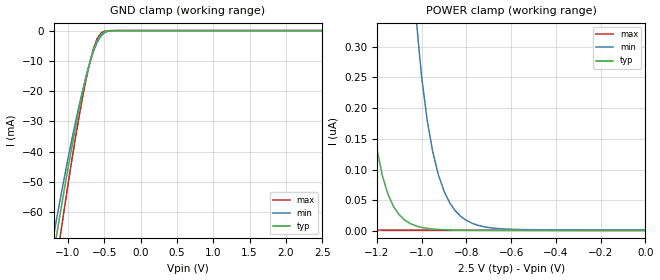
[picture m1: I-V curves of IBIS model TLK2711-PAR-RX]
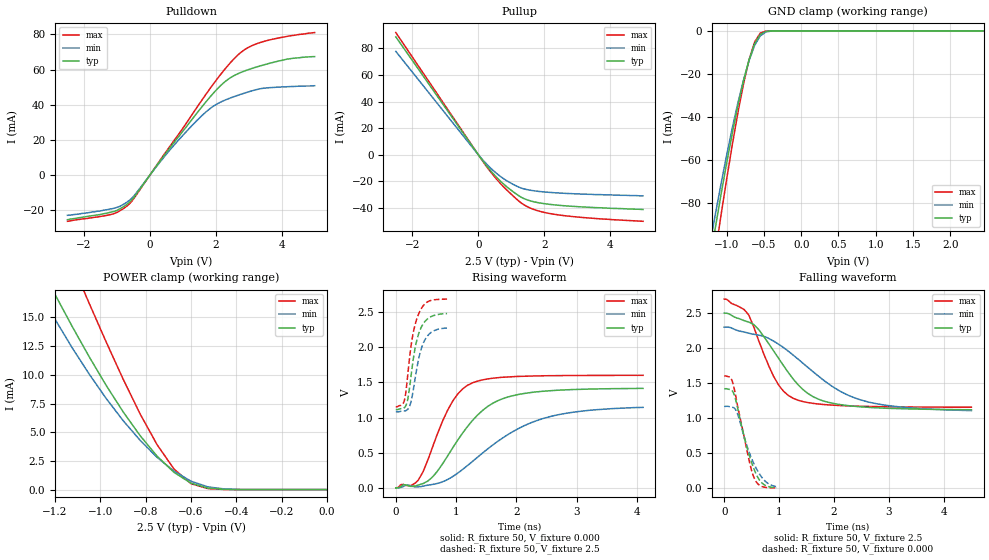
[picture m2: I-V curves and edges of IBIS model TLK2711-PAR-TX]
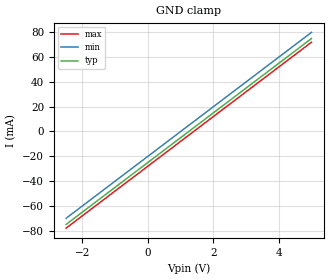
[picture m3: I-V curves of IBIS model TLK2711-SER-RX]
[IBIS ver]   3.2
[File name]   tlk2711.ibs
[File Rev]   0
[Date]   05/17/2001
[Source]   TI
[Notes]   This model is for the TLK2711/TLK2711A SerDes device
[Copyright]   Copyright 2001 Mentor Graphics, Inc.
| (C) COPYRIGHT 1993-2001
| MENTOR GRAPHICS CORPORATION
| ICX STANDARD LIBRARY, ICX PROJECT MODELING,
| ICX CUSTOM MODELING, ICX VENDOR MODEL
| ALL RIGHTS RESERVED.
| THE FOLLOWING ARE TRADEMARKS OR SERVICE MARKS OF
| MENTOR GRAPHICS CORPORATION:ICX (R), ICX STANDARD
| LIBRARY(R), ICX PROJECT MODELING(R), ICX CUSTOM
| MODELING(R), qualityIBIS(TM), MODELVIEWER(TM),  AND MODELEDITOR(TM).
| ALL COPIES OF SOFTWARE, INCLUDING BUT NOT LIMITED TO
| ANY MODIFICATIONS, ENHANCEMENTS OR DERIVATIVE
| WORKS, MUST CONTAIN ALL MENTOR GRAPHICS
| CORPORATION'S NOTICES AND LEGENDS, INCLUDING
| THOSE EMBEDDED IN SOFTWARE AND THOSE AFFIXED
| TO SOFTWARE MEDIUM AND CONTAINER, AS RECEIVED
| FROM MENTOR GRAPHICS CORPORATION
| ALL OTHER BRANDS AND PRODUCT NAMES ARE
| TRADEMARKS OF THEIR RESPECTIVE OWNERS.
| LICENSED SOFTWARE IS THE LICENSE TO USE THE
| ICX STANDARD LIBRARY ICX PROJECT MODELING
| ICX CUSTOM MODELING ICX VENDOR MODEL
|   Component TLK2711
[Component]   TLK2711
[Manufacturer]  TI
[Package]
| variable   typ   min   max
R_pkg   0.0m   0.0m   0.0m
L_pkg   0.0nH   0.0nH   0.0nH
C_pkg   0.0pF   0.0pF   0.0pf
[Pin]   signal_name   model_name   R_pin   L_pin   C_pin
1   VDD   POWER
2   TXD3   TLK2711-PAR-RX
3   TXD4   TLK2711-PAR-RX
4   TXD5   TLK2711-PAR-RX
5   GND   GND
6   TXD6   TLK2711-PAR-RX
7   TXD7   TLK2711-PAR-RX
8   GTX_CLK   TLK2711-PAR-RX
9   VDD   POWER
10   TXD8   TLK2711-PAR-RX
11   TXD9   TLK2711-PAR-RX
12   TXD10   TLK2711-PAR-RX
13   GND   GND
14   TXD11   TLK2711-PAR-RX
15   TXD12   TLK2711-PAR-RX
16   TXD13   TLK2711-PAR-RX
17   TXD14   TLK2711-PAR-RX
18   GND   GND
19   TXD15   TLK2711-PAR-RX
20   TKMSB   TLK2711-PAR-RX
21   LOOPEN   TLK2711-PAR-RX
22   TKLSB   TLK2711-PAR-RX
23   VDD   POWER
24   ENABLE   TLK2711-PAR-RX
25   LCKREFN   TLK2711-PAR-RX
26   PRBSEN   TLK2711-PAR-RX
27   TESTEN   TLK2711-PAR-RX
28   GND   GND
29   RKLSB   TLK2711-PAR-TX
30   RKMSB   TLK2711-PAR-TX
31   RXD15   TLK2711-PAR-TX
32   RXD14   TLK2711-PAR-TX
33   GND   GND
34   RXD13   TLK2711-PAR-TX
35   RXD12   TLK2711-PAR-TX
36   RXD11   TLK2711-PAR-TX
37   RXD10   TLK2711-PAR-TX
38   VDD   POWER
39   RXD9   TLK2711-PAR-TX
40   RXD8   TLK2711-PAR-TX
41   RX_CLK   TLK2711-PAR-TX
42   RXD7   TLK2711-PAR-TX
43   GND   GND
44   RXD6   TLK2711-PAR-TX
45   RXD5   TLK2711-PAR-TX
46   RXD4   TLK2711-PAR-TX
47   RXD3   TLK2711-PAR-TX
48   VDD   POWER
49   RXD2   TLK2711-PAR-TX
50   RXD1   TLK2711-PAR-TX
51   RXD0   TLK2711-PAR-TX
52   GNDA   GND
53   DINRXN   TLK2711-SER-RX
54   DINRXP   TLK2711-SER-RX
55   VDDA   POWER
56   PRE   TLK2711-PAR-RX
57   VDDA   POWER
58   GNDA   GND
59   DOUTTXN   TLK2711-SER-TX
60   DOUTTXP   TLK2711-SER-TX
61   GNDA   GND
62   TXD0   TLK2711-PAR-RX
63   TXD1   TLK2711-PAR-RX
64   TXD2   TLK2711-PAR-RX
[Diff Pin]   inv_pin   vdiff   tdelay_typ tdelay_min tdelay_max
  54   53   200mV   NA   NA   NA
  60   59   1200mV   NA   NA   NA
[Model selector]   TLK2711-SER-TX
TLK2711-SER-TX_05  TLK2711-SER-TX_05
TLK2711-SER-TX_20  TLK2711-SER-TX_20
| Models and submodels in the file (5): TLK2711-PAR-RX (Input), TLK2711-PAR-TX (3-state), TLK2711-SER-RX (Input), TLK2711-SER-TX_05 (3-state), TLK2711-SER-TX_20 (3-state)
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|   Model TLK2711-PAR-RX
[Model]   TLK2711-PAR-RX
Model_type   Input
Polarity   Non-Inverting
Vinl = 0.8
Vinh = 1.7
| C_comp is estimated by modeling group by simulation
C_comp   3.7441pF   3.6871pF   4.0174pF
[Temperature Range]   27   85   -40
[Voltage Range]   2.5V   2.3V   2.7V
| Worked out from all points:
|   GND clamp passes 1 mA (typ) near -0.53 V on its own axis
[GND_clamp]
| voltage   I(typ)   I(min)   I(max)
-2.5V     -288.4mA   -250.7mA   -333.7mA
-1.2V     -74mA      -67.93mA   -83.57mA
-1.15V    -66.63mA   -61.3mA    -75.13mA
-1.1V     -59.4mA    -54.81mA   -66.86mA
-900mV    -32.43mA   -30.56mA   -35.81mA
-750mV    -15.24mA   -15.04mA   -15.99mA
-650mV    -6.415mA   -6.91mA    -6.009mA
-600mV    -3.327mA   -3.931mA   -2.733mA
-550mV    -1.373mA   -1.882mA   -907.2uA
-500mV    -442.8uA   -741.1uA   -217.9uA
-300mV    -1.064uA   -5.027uA   -93.53nA
2.5V      1.177nA    2.08nA     1.12nA
[POWER_clamp]
| voltage   I(typ)   I(min)   I(max)
-2.5V     46.33uA    53.89uA    38.04uA
-1.525V   5.372uA    12.24uA    372.7nA
-1.475V   3.879uA    10.41uA    138.8nA
-1.425V   2.598uA    8.65uA     49.16nA
-1.275V   432.3nA    4.052uA    3.436nA
-1.25V    296.4nA    3.424uA    2.672nA
-1.225V   200.5nA    2.849uA    2.227nA
-1.175V   89.61nA    1.871uA    1.813nA
-1.025V   8.517nA    347.8nA    1.568nA
-950mV    3.456nA    128.4nA    1.536nA
-825mV    1.702nA    24nA       1.489nA
0V        1.177nA    2.005nA    1.192nA
|   Model TLK2711-PAR-TX
[Model]   TLK2711-PAR-TX
Model_type   3-state
Polarity   Non-Inverting
Enable   Active-Low
| Timing test load is based on data sheet information for rise and fall time
Vmeas = 1.5V
Cref  = 3pF
Rref  = 1Mohms
Vref  = 0V
| C_comp is estimated by modeling group by simulation
C_comp   2.0899pF   2.0661pF   2.1142pF
[Temperature Range]   27   85   -40
[Voltage Range]   2.5V   2.3V   2.7V
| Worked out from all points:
|   slope of the pulldown table from 0 to 0.375 V, typ, clamps not added: 38.6 ohm
|   slope of the pullup table from 0 to 0.375 V, typ, clamps not added: 31 ohm
|   GND clamp passes 1 mA (typ) near -0.51 V on its own axis
|   POWER clamp passes 1 mA (typ) near -0.64 V on its own axis
|   rising waveform, R_fixture 50, V_fixture 0.000: 20-80 % time 757ps typ, 1.16ns min, 486ps max; typ from 0 V to 1.42 V
|   rising waveform, R_fixture 50, V_fixture 2.5: 20-80 % time 163ps typ, 170ps min, 159ps max; typ from 1.11 V to 2.48 V
|   falling waveform, R_fixture 50, V_fixture 2.5: 20-80 % time 788ps typ, 1.23ns min, 507ps max; typ from 2.5 V to 1.12 V
|   falling waveform, R_fixture 50, V_fixture 0.000: 20-80 % time 288ps typ, 314ps min, 257ps max; typ from 1.42 V to 0.008 V
[Pulldown]
| voltage   I(typ)   I(min)   I(max)
-2.5V     -25.3mA    -22.8mA    -26.2mA
-1.15V    -20.87mA   -19.05mA   -22.2mA
-925mV    -19.28mA   -17.8mA    -20.41mA
-625mV    -15.5mA    -14.37mA   -16.41mA
650mV     16.54mA    15.22mA    17.47mA
1.625V    39.88mA    34.61mA    43.86mA
2.225V    52.22mA    42.18mA    59.03mA
2.825V    58.83mA    46.34mA    70.64mA
3.125V    60.8mA     48.04mA    73.8mA
3.575V    63.25mA    49.63mA    76.55mA
4.175V    65.94mA    50.25mA    78.88mA
5V        67.36mA    50.81mA    81.01mA
[Pullup]
| voltage   I(typ)   I(min)   I(max)
-2.5V     88.77mA    77.8mA     92.01mA
-25mV     881.6uA    757.4uA    929.9uA
200mV     -6.727mA   -5.695mA   -7.178mA
425mV     -13.52mA   -11.31mA   -14.56mA
725mV     -21.21mA   -17.4mA    -23.16mA
1.025V    -27.36mA   -21.98mA   -30.38mA
1.325V    -32.43mA   -25.4mA    -36.84mA
1.55V     -34.65mA   -26.73mA   -39.98mA
1.775V    -36.03mA   -27.57mA   -42.1mA
2.375V    -38.07mA   -28.86mA   -45.26mA
3.275V    -39.62mA   -29.89mA   -47.65mA
5V        -41.4mA    -31.1mA    -50.3mA
[GND_clamp]
| voltage   I(typ)   I(min)   I(max)
-2.5V     -398.5mA   -366.5mA   -446.5mA
-1.225V   -106.7mA   -99.28mA   -120.4mA
-1.15V    -91.03mA   -84.85mA   -102.7mA
-1.075V   -75.9mA    -70.95mA   -85.44mA
-925mV    -47.65mA   -45.15mA   -52.95mA
-775mV    -23.32mA   -22.97mA   -24.76mA
-700mV    -13.43mA   -13.85mA   -13.42mA
-625mV    -5.934mA   -6.74mA    -5.161mA
-550mV    -1.689mA   -2.34mA    -1.084mA
-475mV    -286.3uA   -539.4uA   -114.6uA
-325mV    -3.039uA   -12.61uA   -323.9nA
2.45V     7.078nA    15.31nA    6.305nA
[POWER_clamp]
| voltage   I(typ)   I(min)   I(max)
-2.475V   71.34mA    69.04mA    72.85mA
-1.275V   19.87mA    17.42mA    26.56mA
-1.2V     16.99mA    14.83mA    23.15mA
-1.125V   14.23mA    12.37mA    19.69mA
-1.05V    11.59mA    10.08mA    16.25mA
-900mV    6.787mA    6.019mA    9.637mA
-750mV    2.917mA    2.814mA    3.917mA
-675mV    1.498mA    1.606mA    1.79mA
-600mV    558.2uA    731uA      514.2uA
-525mV    131uA      233.8uA    82.45uA
-450mV    19.71uA    49.19uA    8.091uA
0V        7.061nA    7.795nA    7.52nA
[Ramp]
| variable   typ   min   max
dV/dt_r 0.8496V/0.756579ns  0.6876V/1.15604ns  0.9612V/0.485909ns
dV/dt_f 0.828V/0.787902ns  0.7152V/1.22754ns  0.9258V/0.506788ns
R_load = 50
[Rising Waveform]
R_fixture = 50
V_fixture = 0.000
V_fixture_min = 0.000
V_fixture_max = 0.000
| time   V(typ)   V(min)   V(max)
0s        0V         0V         0V
369ps     38.81mV    14.16mV    106.4mV
615ps     160.1mV    49.57mV    594.2mV
902ps     512.8mV    138.8mV    1.172V
1.107ns   779mV      261.7mV    1.408V
1.271ns   958.7mV    376.3mV    1.495V
1.681ns   1.237V     655.9mV    1.567V
2.378ns   1.37V      969.7mV    1.594V
2.993ns   1.401V     1.083V     1.6V
4.1ns     1.416V     1.146V     1.602V
[Rising Waveform]
R_fixture = 50
V_fixture = 2.5
V_fixture_min = 2.3
V_fixture_max = 2.7
| time   V(typ)   V(min)   V(max)
0s        1.115V     1.084V     1.155V
136ps     1.138V     1.094V     1.226V
187ps     1.218V     1.11V      1.516V
238ps     1.493V     1.185V     1.925V
272ps     1.723V     1.307V     2.128V
323ps     2.002V     1.571V     2.334V
391ps     2.223V     1.882V     2.5V
459ps     2.341V     2.066V     2.598V
544ps     2.417V     2.182V     2.656V
850ps     2.482V     2.276V     2.687V
[Falling Waveform]
R_fixture = 50
V_fixture = 2.5
V_fixture_min = 2.3
V_fixture_max = 2.7
| time   V(typ)   V(min)   V(max)
0s        2.5V       2.3V       2.7V
450ps     2.371V     2.213V     2.47V
630ps     2.263V     2.185V     2.103V
900ps     1.961V     2.1V       1.596V
1.08ns    1.75V      2.008V     1.385V
1.26ns    1.555V     1.898V     1.282V
1.71ns    1.273V     1.604V     1.203V
2.475ns   1.163V     1.263V     1.17V
3.195ns   1.136V     1.161V     1.161V
4.5ns     1.12V      1.108V     1.157V
[Falling Waveform]
R_fixture = 50
V_fixture = 0.000
V_fixture_min = 0.000
V_fixture_max = 0.000
| time   V(typ)   V(min)   V(max)
0s        1.419V     1.168V     1.602V
104.5ps   1.41V      1.162V     1.584V
161.5ps   1.373V     1.154V     1.49V
237.5ps   1.17V      1.072V     1.202V
351.5ps   776.3mV    764.6mV    774.4mV
465.5ps   448.1mV    490.2mV    356.2mV
551ps     256.8mV    332.9mV    136.6mV
617.5ps   146.4mV    234.5mV    58.44mV
712.5ps   58.08mV    128.9mV    18.2mV
950ps     8.214mV    21.82mV    4.967mV
|   Model TLK2711-SER-RX
[Model]   TLK2711-SER-RX
Model_type   Input
Polarity   Non-Inverting
Vinl = 1.15
Vinh = 1.35
| C_comp is estimated by modeling group by simulation
C_comp   1.3073pF   1.2955pF   1.3193p
[Temperature Range]   27   85   -40
[Voltage Range]   2.5V   2.3V   2.7V
[GND_clamp]
| voltage   I(typ)   I(min)   I(max)
-2.5V     -75mA      -70.04mA   -77.99mA
1.025V    -4.5mA     463uA      -7.488mA
1.55V     6mA        10.96mA    3.012mA
5V        75mA       79.96mA    72.01mA
